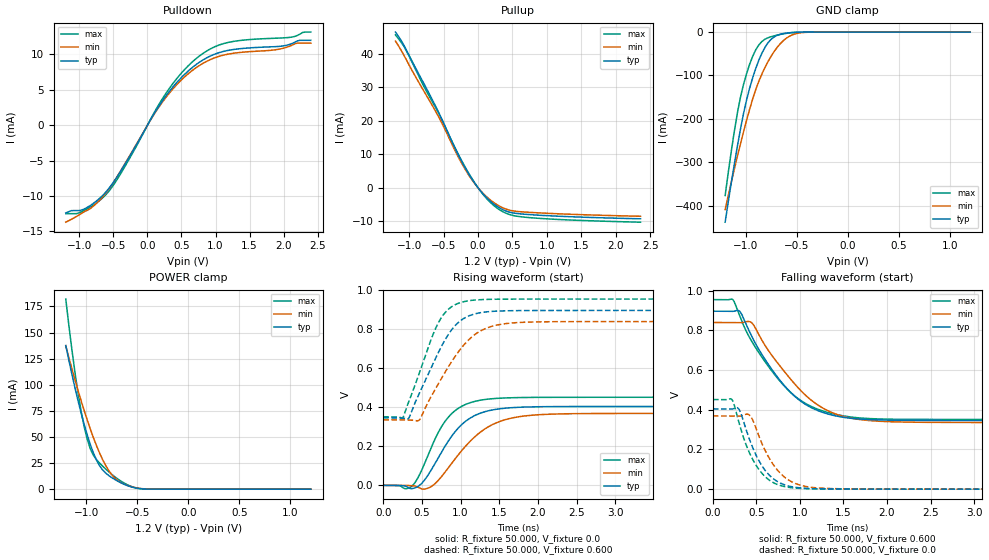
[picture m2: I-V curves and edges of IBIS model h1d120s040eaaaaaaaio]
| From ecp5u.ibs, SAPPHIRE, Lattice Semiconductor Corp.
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|   Model h1d120s040eaaaaaaaio
[Model] h1d120s040eaaaaaaaio
Model_type I/O
Polarity   Non-Inverting
Enable   Active-Low
Vinl =  0.500V
Vinh =  0.700V
Vmeas =  0.600V
Cref =  20.000pF
Rref =  50.000
Vref =  0.600V
C_comp   5.000pF   4.000pF   5.500pF
[Temperature Range]   25.000   0.125k   -40.000
[Voltage Range]   1.200V   1.140V   1.260V
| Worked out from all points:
|   slope of the pulldown table from 0 to 0.18 V, typ, clamps not added: 62.6 ohm
|   slope of the pullup table from 0 to 0.18 V, typ, clamps not added: 44.5 ohm
|   GND clamp passes 1 mA (typ) near -0.54 V on its own axis
|   POWER clamp passes 1 mA (typ) near -0.51 V on its own axis
|   rising waveform, R_fixture 50.000, V_fixture 0.0: 20-80 % time 425ps typ, 526ps min, 357ps max; typ from 0 V to 0.404 V
|   rising waveform, R_fixture 50.000, V_fixture 0.600: 20-80 % time 415ps typ, 493ps min, 342ps max; typ from 0.346 V to 0.897 V
|   falling waveform, R_fixture 50.000, V_fixture 0.600: 20-80 % time 543ps typ, 586ps min, 590ps max; typ from 0.897 V to 0.346 V
|   falling waveform, R_fixture 50.000, V_fixture 0.0: 20-80 % time 261ps typ, 284ps min, 260ps max; typ from 0.404 V to 0 V
[Pulldown]
|Voltage   I(typ)   I(min)   I(max)
-1.2V     -12.39mA   -13.7mA    -12.49mA
-1.04V    -12.05mA   -12.88mA   -12.49mA
-880mV    -11.58mA   -12mA      -11.79mA
-560mV    -8.851mA   -8.925mA   -9.245mA
-280mV    -4.688mA   -4.607mA   -4.974mA
200mV     3.164mA    3.008mA    3.437mA
440mV     6.136mA    5.828mA    6.7mA
680mV     8.315mA    7.89mA     9.126mA
920mV     9.761mA    9.262mA    10.76mA
1.16V     10.53mA    9.999mA    11.64mA
2.08V     11.4mA     11.13mA    12.4mA
2.4V      12mA       11.6mA     13.16mA
[Pullup]
|Voltage   I(typ)   I(min)   I(max)
-1.2V     46.58mA    43.88mA    45.74mA
-1.08V    42.72mA    39.74mA    42.43mA
-1.04V    41.15mA    38.23mA    40.88mA
-800mV    31.67mA    29.37mA    30.83mA
-560mV    22.01mA    20.73mA    21.77mA
-320mV    11.18mA    10.54mA    11.37mA
-160mV    4.974mA    4.595mA    5.205mA
40mV      -1.043mA   -938.5uA   -1.131mA
240mV     -5.059mA   -4.599mA   -5.498mA
440mV     -7.189mA   -6.594mA   -7.881mA
640mV     -7.846mA   -7.203mA   -8.71mA
2.36V     -9.281mA   -8.526mA   -10.29mA
[GND_clamp]
|Voltage   I(typ)   I(min)   I(max)
-1.2V     -438mA     -409mA     -376.5mA
-1.14V    -347.3mA   -346mA     -274.9mA
-1.08V    -262.9mA   -286.2mA   -185.9mA
-1.05V    -223.7mA   -257.6mA   -150mA
-990mV    -156.1mA   -203.2mA   -95.66mA
-930mV    -105mA     -153.7mA   -55.58mA
-870mV    -64.74mA   -113.2mA   -29.56mA
-810mV    -35.2mA    -81.56mA   -16.45mA
-720mV    -11.09mA   -44.69mA   -8.691mA
-600mV    -2.287mA   -13.94mA   -2.904mA
-450mV    -166.2uA   -1.247mA   -164.1uA
1.2V      0A         0A         0A
[POWER_clamp]
|Voltage   I(typ)   I(min)   I(max)
-1.2V     137.6mA    137.3mA    182.1mA
-1.14V    110.1mA    115.3mA    133.6mA
-1.08V    84.76mA    94.63mA    92.15mA
-1.02V    62.11mA    75.36mA    59.94mA
-990mV    52mA       66.3mA     47.89mA
-930mV    34.81mA    49.51mA    32.55mA
-870mV    22.62mA    34.86mA    25.07mA
-780mV    13.14mA    18.01mA    16.74mA
-720mV    9.284mA    10.72mA    11.88mA
-600mV    3.553mA    3.709mA    4.373mA
-450mV    294.8uA    471.6uA    256.4uA
1.2V      0A         0A         0A
[Ramp]
| variable   typ   min   max
dV/dt_r 0.243/0.432n   0.221/0.528n   0.271/0.362n
dV/dt_f 0.266/0.570n   0.247/0.546n   0.295/0.639n
R_load = 50.000
[Rising Waveform]
R_fixture= 50.000
V_fixture= 0.0
V_fixture_min= 0.0
V_fixture_max= 0.0
|time   V(typ)   V(min)   V(max)
0s        0V         0V         0V
366ps     -16.76mV   -1.233mV   -5.533mV
611ps     72.67mV    -8.232mV   184.8mV
755ps     171.5mV    45.69mV    301.8mV
910ps     265.7mV    126.1mV    376.8mV
1.111ns   341.7mV    221.1mV    422.1mV
1.351ns   381.5mV    298.6mV    441.9mV
1.716ns   399.6mV    349.3mV    449.8mV
2.281ns   403.9mV    366.3mV    451.4mV
10ns      404.4mV    368.9mV    451.5mV
[Rising Waveform]
R_fixture= 50.000
V_fixture= 0.600
V_fixture_min= 0.571
V_fixture_max= 0.631
|time   V(typ)   V(min)   V(max)
0s        346.3mV    335.9mV    351.2mV
256ps     344.7mV    335.8mV    348.9mV
334ps     346.7mV    334.9mV    433.1mV
470ps     475mV      336.7mV    579.4mV
765ps     721.7mV    557mV      867.8mV
922ps     815.9mV    656.9mV    924.6mV
1.1ns     867.6mV    744.5mV    946mV
1.401ns   891.7mV    815.1mV    953.8mV
1.911ns   896.3mV    837.3mV    954.9mV
10ns      896.6mV    839.6mV    955mV
[Falling Waveform]
R_fixture= 50.000
V_fixture= 0.600
V_fixture_min= 0.571
V_fixture_max= 0.631
|time   V(typ)   V(min)   V(max)
0s        896.6mV    839.7mV    955mV
232ps     895.8mV    839.6mV    953.5mV
313ps     893.8mV    838.7mV    867.3mV
439ps     776.3mV    840.6mV    750.1mV
698ps     590.3mV    661.8mV    583.3mV
957ps     461.4mV    521.4mV    463.5mV
1.244ns   389.5mV    413.4mV    396.5mV
1.568ns   357.9mV    359.3mV    364.5mV
2.498ns   346.4mV    336.6mV    351.3mV
10ns      346.3mV    335.9mV    351.2mV
[Falling Waveform]
R_fixture= 50.000
V_fixture= 0.0
V_fixture_min= 0.0
V_fixture_max= 0.0
|time   V(typ)   V(min)   V(max)
0s        404.4mV    368.9mV    451.6mV
224ps     403.8mV    368.9mV    448.1mV
303ps     400.3mV    367.9mV    330.3mV
420ps     251.2mV    372.9mV    182.8mV
528ps     143.5mV    267.8mV    99.44mV
638ps     75.01mV    163.1mV    48.76mV
765ps     32.66mV    84.28mV    19.74mV
925ps     10.83mV    32.74mV    6.221mV
1.656ns   425uV      917.4uV    504uV
10ns      0V         0V         0V
